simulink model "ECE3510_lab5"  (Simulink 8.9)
settings: Solver=FixedStepDiscrete  StartTime=0.0  StopTime=Inf  FixedStep=Ts  RelTol=1e-3  EnableMultiTasking=on
PostLoadFcn:
  | , if any(exist('dsrtsu_mdlpostloadfcn', 'file') == [2, 3, 6]), try dsrtsu_mdlpostloadfcn('Execute', bdroot); catch fprintf('Error in PostLoadFcn (dsrtsu_mdlpostloadfcn) for model "%s":
  |  %s
  | ', bdroot, lasterr); end, end,
InitFcn:
  | Ts=1e-4;
  | nd = 30;
undefined symbols (not defined in the file or in its folder): DiscIntNeverNeededParam
libraries: rtilib1104 x4

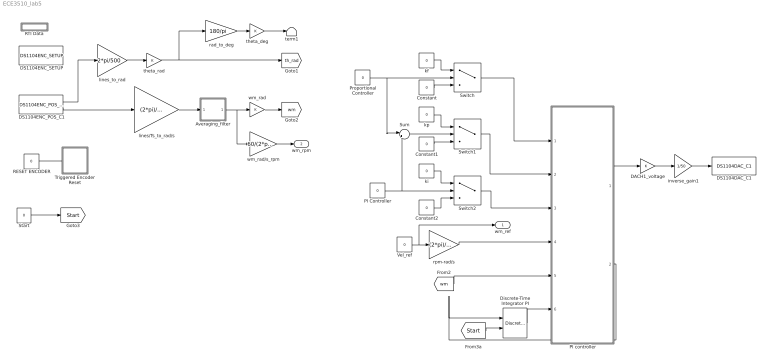
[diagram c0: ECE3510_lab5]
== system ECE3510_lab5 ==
  Averaging_filter : Subsystem
  Constant : Constant  Value=0
  Constant1 : Constant  Value=0
  Constant2 : Constant  Value=0
  DACH1_voltage : Gain  OutMin=-25  OutMax=25
  DS1104DAC_C1 : rtilib1104/DS1104 MASTER PPC/DS1104DAC_C1  ChannelNo=1  InitValue=0  TermMode=0  TermValue=0  Reserved1=[]  Reserved2=[]  Reserved3=[]  Reserved4=[]  DialogFcn=gui1104dac  UnitName={ 'DS1104DAC_C'}  UnitValues={ 1 }  DSProperties=struct('RTI',struct('Version',uint32(1),'BlockType',struct('isSLSource',uint8(0),'isSLSink',uint8(1),'isHWSource',uint8(0),'isHWSink',uint8(1),'isSetup',uint8(0),'isInline',uint8(1),'isNonInline',uint8(0),'isInterrupt',uint8(0),'isChannelwise',uint8(1)),'IOBoardType','DS1104MASTER','UnitType','DAC','Identifier','DAC','DialogType','ML','BlockSet','NONE','SlaveProcessor','NONE'))
  DS1104ENC_POS_C1 : rtilib1104/DS1104 MASTER PPC/DS1104ENC_POS_C1  ChannelNo=1  PosValue=0  Reserved1=[]  Reserved2=[]  Reserved3=[]  Reserved4=[]  DialogFcn=gui1104enc_pos  UnitName={'DS1104ENC_POS_C'}  UnitValues={ 1 }  DSProperties=struct('RTI',struct('Version',uint32(1),'BlockType',struct('isSLSource',uint8(1),'isSLSink',uint8(0),'isHWSource',uint8(1),'isHWSink',uint8(0),'isSetup',uint8(0),'isInline',uint8(1),'isNonInline',uint8(0),'isInterrupt',uint8(0),'isChannelwise',uint8(1)),'IOBoardType','DS1104MASTER','UnitType','ENC','Identifier','ENCPOSCH','DialogType','ML','BlockSet','NONE','SlaveProcessor','NONE'))
  DS1104ENC_SETUP : rtilib1104/DS1104 MASTER PPC/DS1104ENC_SETUP  Reserved1=[]  Reserved2=[]  Reserved3=[]  Reserved4=[]  DialogFcn=gui1104enc_setup  UnitName={'DS1104ENC_SETUP'}  UnitValues={ [] }  DSProperties=struct('RTI',struct('Version',uint32(1),'BlockType',struct('isSLSource',uint8(0),'isSLSink',uint8(0),'isHWSource',uint8(0),'isHWSink',uint8(0),'isSetup',uint8(0),'isInline',uint8(1),'isNonInline',uint8(0),'isInterrupt',uint8(0),'isChannelwise',uint8(0)),'IOBoardType','DS1104MASTER','UnitType','ENC','Identifier','ENCSETUP','DialogType','ML','BlockSet','NONE','SlaveProcessor','NONE'))
  Discrete-Time Integrator PI : DiscreteIntegrator  ExternalReset=rising  SampleTime=-1  ICPrevOutput=DiscIntNeverNeededParam  ICPrevScaledInput=DiscIntNeverNeededParam
  PI Controller : Constant  Value=0
  PI controller : MATLAB Function  TreatAsAtomicUnit=on
  Proportional Controller : Constant  Value=0
  RESET ENCODER : Constant  Value=0
  RTI Data : Subsystem  Tag=struct('RTIDataServer',struct('RTIDataServerVs','2','RTIModelDescription','struct(''main'',''ECE3510_lab5'',''sub'','''',''isMp'',0)'))  LoadFcn="if exist('rtidc'), try,  rtidc('DataHostBlockClbLoad', gcbh); catch, disp(['Warning: ''LoadFcn'' for RTI Data block failed: ' lasterr]); end, end,"
  Start : Constant  Value=0
  Sum : Sum  Inputs=|++
  Switch : Switch  Threshold=0.5
  Switch1 : Switch  Threshold=0.5
  Switch2 : Switch  Threshold=0.5
  Triggered Encoder Reset : Subsystem  TreatAsAtomicUnit=on
  Vel_ref : Constant  Value=0
  inverse_gain1 : Gain  Gain=1/50
  kf : Constant  Value=0
  ki : Constant  Value=0
  kp : Constant  Value=0
  lines/Ts_to_rad/s : Gain  Gain=(2*pi)/(500*Ts)
  lines_to_rad : Gain  Gain=2*pi/500
  rad_to_deg : Gain  Gain=180/pi
  rpm-rad/s : Gain  Gain=(2*pi)/60
  term1 : Terminator
  theta_deg : Gain
  theta_rad : Gain
  wm_rad : Gain
  wm_rad/s_rpm : Gain  Gain=60/(2*pi)
  wm_ref : Outport
  wm_rpm : Outport  Port=2
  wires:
  DS1104ENC_POS_C1/2 -> lines/Ts_to_rad/s/1
  lines/Ts_to_rad/s/1 -> Averaging_filter/1(in)
  wm_rad/1 -> [wm]
  DACH1_voltage/1 -> inverse_gain1/1
  inverse_gain1/1 -> DS1104DAC_C1/1
  DS1104ENC_POS_C1/1 -> lines_to_rad/1
  lines_to_rad/1 -> theta_rad/1
  theta_rad/1 -> rad_to_deg/1, [th_rad]
  PI controller/1(u) -> DACH1_voltage/1
  Vel_ref/1 -> wm_ref/1, rpm-rad/s/1
  Start/1 -> [Start]
  [Start] -> Discrete-Time Integrator PI/2
  PI controller/2(die) -> Discrete-Time Integrator PI/1
  rpm-rad/s/1 -> PI controller/4(r)
  Discrete-Time Integrator PI/1 -> PI controller/6(ie)
  [wm] -> PI controller/5(y)
  rad_to_deg/1 -> theta_deg/1
  theta_deg/1 -> term1/1
  RESET ENCODER/1 -> Triggered Encoder Reset/Trigger
  Constant/1 -> Switch/3
  Proportional Controller/1 -> Switch/2, Sum/1
  kf/1 -> Switch/1
  Switch/1 -> PI controller/1(kf)
  kp/1 -> Switch1/1
  Constant1/1 -> Switch1/3
  Switch1/1 -> PI controller/2(kp)
  ki/1 -> Switch2/1
  PI Controller/1 -> Sum/2, Switch2/2
  Constant2/1 -> Switch2/3
  Switch2/1 -> PI controller/3(ki)
  Averaging_filter/1(out) -> wm_rad/s_rpm/1, wm_rad/1
  wm_rad/s_rpm/1 -> wm_rpm/1
  Sum/1 -> Switch1/2

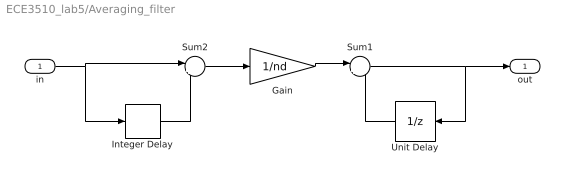
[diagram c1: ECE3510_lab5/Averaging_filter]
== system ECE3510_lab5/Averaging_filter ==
  in : Inport
  Gain : Gain  Gain=1/nd
  Integer Delay : Delay  DelayLength=nd
  Sum1 : Sum  Inputs=|++
  Sum2 : Sum  Inputs=|+-
  Unit Delay : UnitDelay  SampleTime=Ts
  out : Outport
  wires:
  Sum2/1 -> Gain/1
  in/1 -> Sum2/1, Integer Delay/1
  Sum1/1 -> out/1, Unit Delay/1
  Gain/1 -> Sum1/1
  Unit Delay/1 -> Sum1/2
  Integer Delay/1 -> Sum2/2

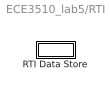
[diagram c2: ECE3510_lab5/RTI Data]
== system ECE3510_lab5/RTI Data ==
  RTI Data Store : Subsystem  Tag=struct('private',struct('version',struct('dsVer',uint32(2),'dsVerCreation',uint32(2),'RTI',struct('ver','6.9','type','RTI1104')),'access',struct('type','Model','isPerm',1,'created',['22-Jan-2015 12:58:17'],'modified',['14-Feb-2019 16:28:51'],'location','')),'public',struct('main',struct('data',[]),'sub',struct('name',{{'ECE3510_lab5'}},'data',{{struct('TH',struct('thTaskInfo',struct('taskType',{'T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

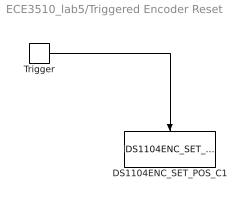
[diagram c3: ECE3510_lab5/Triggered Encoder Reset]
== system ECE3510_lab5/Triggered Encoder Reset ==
  Trigger : TriggerPort  TriggerType=either  VariantControl=Variant  ShowOutputPort=on
  DS1104ENC_SET_POS_C1 : rtilib1104/DS1104 MASTER PPC/DS1104ENC_SET_POS_C1  ChannelNo=1  PosValue=0  Reserved1=[]  Reserved2=[]  Reserved3=[]  Reserved4=[]  DialogFcn=gui1104enc_set_pos  UnitName={'DS1104ENC_SET_POS_C'}  UnitValues={ 1 }  DSProperties=struct('RTI',struct('Version',uint32(1),'BlockType',struct('isSLSource',uint8(0),'isSLSink',uint8(1),'isHWSource',uint8(0),'isHWSink',uint8(1),'isSetup',uint8(0),'isInline',uint8(1),'isNonInline',uint8(0),'isInterrupt',uint8(0),'isChannelwise',uint8(1)),'IOBoardType','DS1104MASTER','UnitType','ENC','Identifier','ENCRESET','DialogType','ML','BlockSet','NONE','SlaveProcessor','NONE'))
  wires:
  Trigger/1 -> DS1104ENC_SET_POS_C1/Trigger

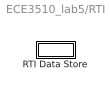
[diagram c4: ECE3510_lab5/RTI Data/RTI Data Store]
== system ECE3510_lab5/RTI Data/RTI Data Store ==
  RTI Data Store : Subsystem

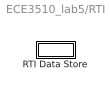
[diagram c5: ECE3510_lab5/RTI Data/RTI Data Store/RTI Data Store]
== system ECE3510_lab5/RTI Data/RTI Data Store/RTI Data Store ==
  RTI Data Store : Subsystem

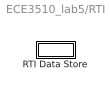
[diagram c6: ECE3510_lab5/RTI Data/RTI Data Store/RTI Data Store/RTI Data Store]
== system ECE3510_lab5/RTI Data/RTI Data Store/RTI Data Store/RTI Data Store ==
  RTI Data Store : Subsystem

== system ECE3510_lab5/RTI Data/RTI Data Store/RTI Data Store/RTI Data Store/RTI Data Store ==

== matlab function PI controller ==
function [u,die] =  PID (kf,kp,ki,r,y,ie)
%
umax=25;  % maximum voltage
%
u=kf*kp*r-kp*y+ki*ie;
die=r-y;
if abs(u)>umax;u=umax*sign(u);end;
